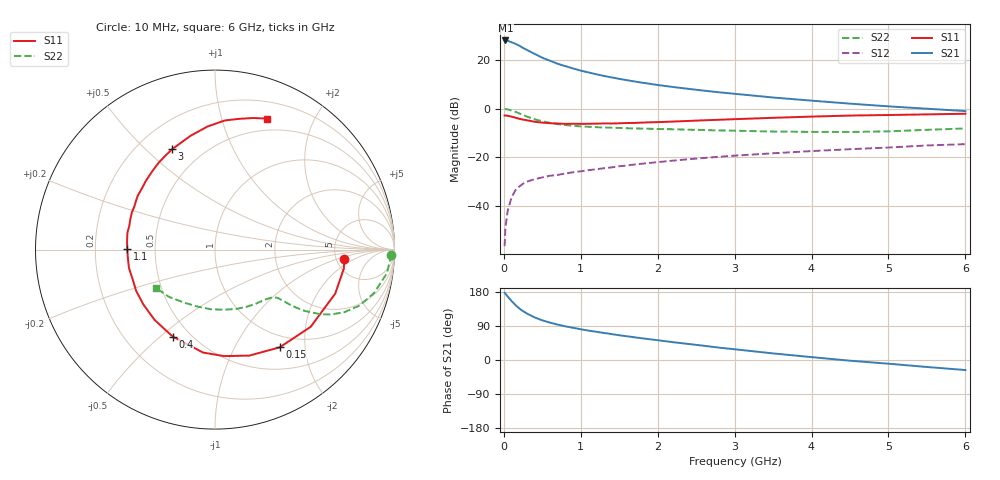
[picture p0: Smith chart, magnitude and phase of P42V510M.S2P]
! SIEMENS Small Signal Semiconductors
! BFP182
! Si NPN RF Bipolar Junction Transistor in SOT143
! VCE = 2.5 V  IC = 10 mA
! Common Emitter S-Parameters:  March  1996
# GHz  S  MA  R  50
!  f  S11  S21  S12  S22
! GHz  MAG  ANG  MAG  ANG  MAG  ANG  MAG  ANG
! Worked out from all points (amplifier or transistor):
!   36 points, 10 MHz to 6 GHz, reference 50 ohm
!   highest |S21| = 28.0 dB at 20 MHz (marker M1)
!   |S21| within 3 dB of that: start of sweep to 246.4 MHz
!   unconditionally stable (mu >= 1): 1.138 GHz to 5.427 GHz
!   at 250 MHz: K = 0.34, MSG = 27.9 dB, |S12| = -30.8 dB
!   at 1.4 GHz: K = 1.09, MAG = 16.6 dB, |S12| = -24.1 dB
!   at 6 GHz: K = 0.94, MSG = 6.8 dB, |S12| = -14.6 dB
!   lowest NFmin = 1.50 dB at 450 MHz
!   S11 on the Smith chart (normalised r, x): 10 MHz: 5.93, -1.29; 150 MHz: 0.81, -1.54; 400 MHz: 0.40, -0.55; 1.1 GHz: 0.34, +0.01; 3 GHz: 0.34, +0.61; 6 GHz: 0.37, +1.41
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0.01  0.723 -4.1  24.86 177.5  0.0015 83.9  0.981 -1.6
0.02  0.7256 -8.4  25.16 175.3  0.0035 87.5  0.979 -3.1
0.05  0.7132 -20.1  24.77 167.4  0.008 83.8  0.9663 -7.9
0.1  0.6851 -38.9  23.15 155.9  0.015 70.4  0.9193 -15.2
0.15  0.653 -56.5  21.54 145.3  0.0211 64.4  0.8634 -21.2
0.2  0.6209 -72.0  19.66 136.2  0.0252 58.5  0.7995 -25.9
0.25  0.5956 -85.1  17.67 128.9  0.0287 54.5  0.7406 -29.2
0.3  0.5775 -96.6  16.09 122.7  0.0317 51.1  0.6891 -31.5
0.4  0.5389 -115.9  13.29 112.3  0.0356 47.6  0.6066 -34.3
0.5  0.5165 -130.7  11.13 104.7  0.0387 44.5  0.5494 -35.7
0.6  0.5028 -142.5  9.629 98.6  0.0419 43.8  0.5115 -36.4
0.7  0.4958 -152.4  8.355 93.4  0.0436 43.7  0.4823 -36.8
0.9  0.4903 -168.1  6.7 85.0  0.0495 44.1  0.4453 -37.5
1.1  0.4894 179.3  5.547 77.6  0.0545 44.6  0.4243 -39.0
1.3  0.497 169.1  4.701 71.4  0.0598 44.6  0.4108 -40.8
1.6  0.5073 156.0  3.846 62.6  0.068 44.6  0.3964 -44.3
2.2  0.5434 135.0  2.785 47.0  0.0856 43.2  0.3773 -53.5
3  0.6084 113.1  2.019 28.3  0.1085 38.6  0.3523 -69.5
3.5  0.6487 102.1  1.696 17.4  0.1213 34.9  0.3392 -81.2
4.5  0.7215 85.7  1.268 -1.8  0.147 27.6  0.3322 -107.7
5.5  0.763 73.9  0.998 -18.4  0.1756 20.2  0.3679 -134.4
6  0.7863 68.2  0.892 -26.5  0.1868 15.4  0.3925 -147.0
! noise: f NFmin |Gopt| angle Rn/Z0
0.45  1.5  0.26  43  0.28
0.9  1.6  0.24  87  0.22
1.8  2.1  0.2  170  0.2
